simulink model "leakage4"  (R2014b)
settings: Solver=ode45  StartTime=0.0  StopTime=10.0  RelTol=1e-3
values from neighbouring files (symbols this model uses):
  ampl1 = 1e-4    (= 0.0001)    [ad_test_2.m]    (also in ad_test_3.m; DA_wandler_spektr_1.m = 1; DA_wandler_spektr_2.m = 1; fourier_reihe1.m = 5)
  ampl2 = 1e-5    (= 1e-05)    [ad_test_2.m]    (also in ad_test_3.m; DA_wandler_spektr_1.m = 1; DA_wandler_spektr_2.m = 1; fourier_reihe1.m = 12)
  fsig1 = 100.5    [leakage_3.m]    (also in leakage_4.m; zero_padd1.m = 100; zero_padd2.m = 100; zero_padd3.m = 100)
  fsig2 = 150.3    [leakage_3.m]    (also in leakage_4.m; zero_padd1.m = ',num2str(fsig2),' Hz und N = ',     num2str(N),' bzw. nfft ; zero_padd2.m = ',num2str(fsig2),' Hz und N = ',     num2str(N),' bzw. nfft ; zero_padd3.m = ',num2str(fsig2),' Hz und N = ',     num2str(N),' bzw. nfft )
  N = 4*1024    (= 4096)    [ad_test_12.m]    (also in ad_test_2.m; ad_test_3.m; DA_wandler_spektr_1.m = 1000; DA_wandler_spektr_2.m = 1024)
  noise = 2    [leakage_4.m]    (also in zero_padd3.m = 0)
  phi1 = pi/3    (= 1.0471975512)    [fourier_reihe1.m]    (also in fourier_reihe2.m; leakage_3.m; leakage_4.m; mehrdeutigkeit_1.m = 3.14159265359)
  phi2 = pi/4    (= 0.785398163397)    [fourier_reihe1.m]    (also in fourier_reihe2.m; leakage_3.m = 0.628318530718; leakage_4.m = 0.628318530718; mehrdeutigkeit_1.m = 3.14159265359)
  pw = sum(hanning(N).^2)/N    [leakage_2.m]    (also in leakage_3.m; leakage_4.m; welch_1.m = sum(hamming(nfft).^2)/nfft; zero_padd2.m = sum(hamming(N).^2)/N)
  Ts = 1/fs    (= 0.00025)    [abtast_rate_1.m]    (also in ad_test_12.m = 0.0009765625; ad_test_2.m = 0.00048828125; ad_test_3.m = 0.00048828125; DA_wandler_spektr_1.m = 0.01)
undefined symbols (not defined in the file or in its folder): get
libraries: dspspect3 x2, dspstat3 x2, dspsigops x2, dspsnks4 x1

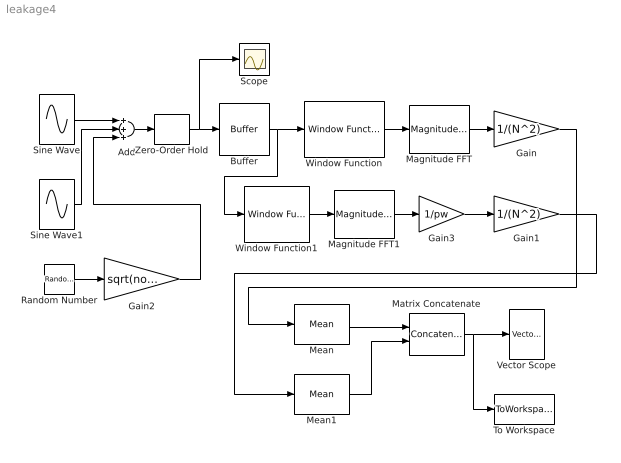
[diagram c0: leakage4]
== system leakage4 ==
  Add : Sum  Inputs=+++
  Buffer : Buffer  N=N  TreatMby1Signals=One channel
  Gain : Gain  Gain=1/(N^2)
  Gain1 : Gain  Gain=1/(N^2)
  Gain2 : Gain  Gain=sqrt(noise)
  Gain3 : Gain  Gain=1/pw
  Magnitude FFT : dspspect3/Magnitude FFT  mag_or_magsq=Magnitude squared  FFTImplementation=Auto  fftLenInherit=on  fftsize=256  WrapInput=on
  Magnitude FFT1 : dspspect3/Magnitude FFT  mag_or_magsq=Magnitude squared  FFTImplementation=Auto  fftLenInherit=on  fftsize=256  WrapInput=on
  Matrix Concatenate : Concatenate  Mode=Multidimensional array  ConcatenateDimension=2
  Mean : dspstat3/Mean  run=on  reset_popup=None  directionMode=Each column  dimension=1  treatSBRowAsCol=on  roiEnable=off  roiType=Rectangles  roiPortion=Entire ROI  roiOutput=Individual statistics for each ROI  roiFlag=off  outputDataTypeStr=Inherit: Same as accumulator  outputLastDataTypeStr=Inherit: Same as accumulator  outputMin=[]  outputMax=[]  roundingMode=Floor  overflowMode=off
  Mean1 : dspstat3/Mean  run=on  reset_popup=None  directionMode=Each column  dimension=1  treatSBRowAsCol=on  roiEnable=off  roiType=Rectangles  roiPortion=Entire ROI  roiOutput=Individual statistics for each ROI  roiFlag=off  outputDataTypeStr=Inherit: Same as accumulator  outputLastDataTypeStr=Inherit: Same as accumulator  outputMin=[]  outputMax=[]  roundingMode=Floor  overflowMode=off
  Random Number : RandomNumber  SampleTime=0
  Scope : Scope
  Sine Wave : Sin  Amplitude=ampl1  Frequency=2*pi*fsig1  Phase=phi1  SampleTime=0
  Sine Wave1 : Sin  Amplitude=ampl2  Frequency=2*pi*fsig2  Phase=phi2  SampleTime=0
  To Workspace : ToWorkspace  VariableName=Y  SampleTime=-1
  Vector Scope : dspsnks4/Vector Scope  ScopeProperties=on  Domain=Frequency  HorizSpan=1  DisplayProperties=off  AxisGrid=on  Memory=off  FrameNumber=on  AxisLegend=off  AxisZoom=off  OpenScopeAtSimStart=on  OpenScopeImmediately=off  FigPos=get(0,'defaultfigureposition')  AxisProperties=off  XUnits=Hertz  XRange=[0...Fs]  InheritXIncr=on  XIncr=1  XLabel=Time  XLimit=Auto  XMin=0  XMax=1  XStart=0  YUnits=dB  YLabel=Leistung in dB  LineProperties=off  XAxisParamsVer=6.9
  Window Function : dspsigops/Window Function  winmode=Apply window to input  wintype=Boxcar  sampmode=Continuous  samptime=1  N=64  Rs=50  beta=10  winsamp=Symmetric  UserWindow=fenster  OptParams=on  UserParams={'symmetric'}  RowConvenienceOn=on  dataType=double  isSigned=on  wordLen=16  udDataType=sfix(16)  fracBitsMode=Best precision  numFracBits=15  roundingMode=Floor  overflowMode=off  numSidelobes=4  sidelobeLevel=-30
  Window Function1 : dspsigops/Window Function  winmode=Apply window to input  wintype=Hanning  sampmode=Continuous  samptime=1  N=64  Rs=50  beta=10  winsamp=Symmetric  UserWindow=fenster  OptParams=on  UserParams={'symmetric'}  RowConvenienceOn=on  dataType=double  isSigned=on  wordLen=16  udDataType=sfix(16)  fracBitsMode=Best precision  numFracBits=15  roundingMode=Floor  overflowMode=off  numSidelobes=4  sidelobeLevel=-30
  Zero-Order Hold : ZeroOrderHold  SampleTime=Ts
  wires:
  Zero-Order Hold/1 -> Scope/1, Buffer/1
  Buffer/1 -> Window Function1/1, Window Function/1
  Magnitude FFT/1 -> Gain/1
  Window Function/1 -> Magnitude FFT/1
  Magnitude FFT1/1 -> Gain3/1
  Gain1/1 -> Mean1/1
  Gain/1 -> Mean/1
  Matrix Concatenate/1 -> To Workspace/1, Vector Scope/1
  Add/1 -> Zero-Order Hold/1
  Sine Wave/1 -> Add/1
  Sine Wave1/1 -> Add/2
  Random Number/1 -> Gain2/1
  Gain2/1 -> Add/3
  Mean/1 -> Matrix Concatenate/1
  Mean1/1 -> Matrix Concatenate/2
  Window Function1/1 -> Magnitude FFT1/1
  Gain3/1 -> Gain1/1
